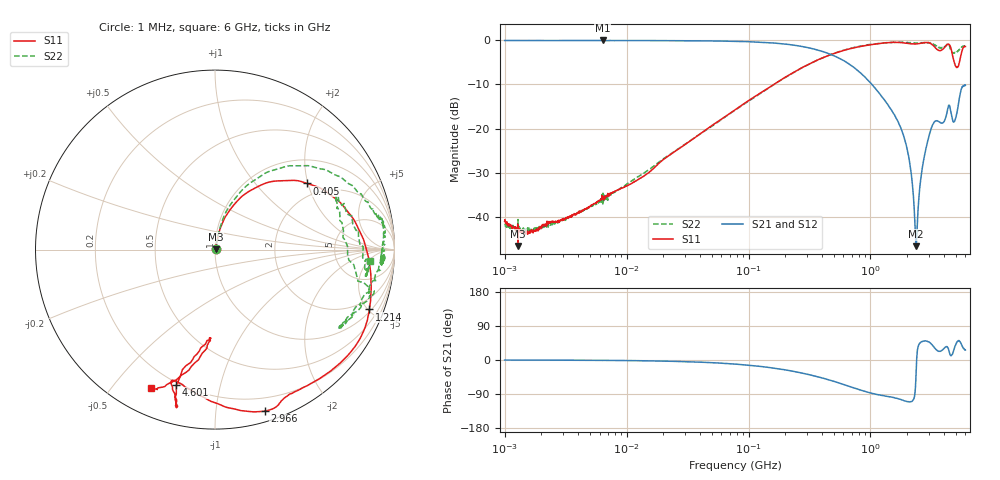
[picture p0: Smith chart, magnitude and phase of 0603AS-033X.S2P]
!s-Parameter Generated by FASTRON Sdn. Bhd.
!FASTRON P/N : 0603AS-033J
!Keysight Technologies: E5071C_MY46733604_B.14.02
!Date: Thu Nov 23 10:55:39 2023
!Version  :Rev01  Thu Nov 23 10:55:39 2023
!Data & Calibration Information:
!Freq  S11:SOLT2(ON)  S21:SOLT2(ON)  S12:SOLT2(ON)  S22:SOLT2(ON)
!PortZ  Port1:50+j0  Port2:50+j0
!When reading reference impedance value at option line is always used.
! Remarks : This data is being provided solely for informational purposes.
# Hz S dB R 50
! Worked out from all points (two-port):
!   1601 points, 1 MHz to 6 GHz, reference 50 ohm
!   highest |S21| = -0.04 dB at 6.378 MHz (marker M1); lowest = -46.6 dB at 2.365 GHz (marker M2)
!   |S21| within 3 dB of the highest: start of sweep to 455.5 MHz
!   lowest |S11| = -46.5 dB at 1.288 MHz (marker M3), VSWR 1.01, Z = 50.4 + j0.216 ohm
!   |S11| at or under -10 dB: start of sweep to 160.5 MHz
!   |S22| runs from -43.8 to -0.4 dB; largest |S21 - S12| = 0.0071
!   S11 on the Smith chart (normalised r, x): 1 MHz: 1.02, +0.01; 405 MHz: 1.61, +1.98; 1.214 GHz: 1.13, -5.11; 2.966 GHz: 0.09, -1.35; 4.601 GHz: 0.19, -0.74; 6 GHz: 0.11, -0.63
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1000000  -40.94 21.6  -0.06 -0.1  -0.07 -0.1  -41.51 22.9
1287650  -46.53 27.0  -0.07 -0.1  -0.05 -0.2  -40.54 15.3
4277066  -38.73 58.3  -0.07 -0.6  -0.06 -0.6  -38.76 58.8
6378092  -35.78 69.3  -0.04 -1.0  -0.09 -1.0  -37.29 69.7
1.823719e7  -27.94 76.9  -0.08 -2.7  -0.09 -2.6  -27.63 75.7
7.757876e7  -15.74 74.1  -0.23 -10.8  -0.24 -10.7  -15.81 76.0
3.307917e8  -5.07 43.7  -1.86 -40.4  -1.86 -40.4  -5.12 53.2
4.050112e8  -3.98 35.6  -2.54 -47.6  -2.53 -47.6  -3.99 47.8
7.448382e8  -1.65 4.4  -6.32 -74.5  -6.31 -74.5  -1.56 25.8
1.214289e9  -0.69 -21.2  -12.43 -93.1  -12.45 -93.1  -0.67 11.0
1.414819e9  -0.51 -27.7  -14.94 -96.9  -14.95 -96.9  -0.51 9.3
1.971195e9  -0.66 -50.2  -23.88 -109.4  -23.89 -109.2  -0.56 2.6
2.365139e9  -0.82 -63.7  -46.56 -35.1  -46.58 -35.1  -0.67 -4.7
2.658144e9  -0.61 -67.6  -28.89 48.7  -28.87 48.7  -0.64 -4.4
2.965799e9  -0.53 -72.9  -22.49 48.3  -22.46 48.4  -0.55 -4.1
3.340973e9  -1.46 -91.6  -18.47 32.3  -18.45 32.2  -1.04 -15.5
3.806705e9  -2.27 -108.4  -18.69 24.1  -18.69 23.9  -1.79 -31.7
4.292686e9  -0.89 -103.7  -15.58 33.3  -15.60 33.2  -0.93 -16.9
4.601007e9  -2.12 -105.9  -16.82 11.6  -16.84 11.5  -2.62 -2.6
5.076665e9  -6.16 -93.5  -16.74 45.0  -16.76 45.0  -2.74 22.3
5.692222e9  -1.95 -109.7  -10.51 34.8  -10.52 34.8  -1.36 -7.0
6e9  -1.42 -114.7  -10.18 26.3  -10.18 26.4  -1.27 -4.3
